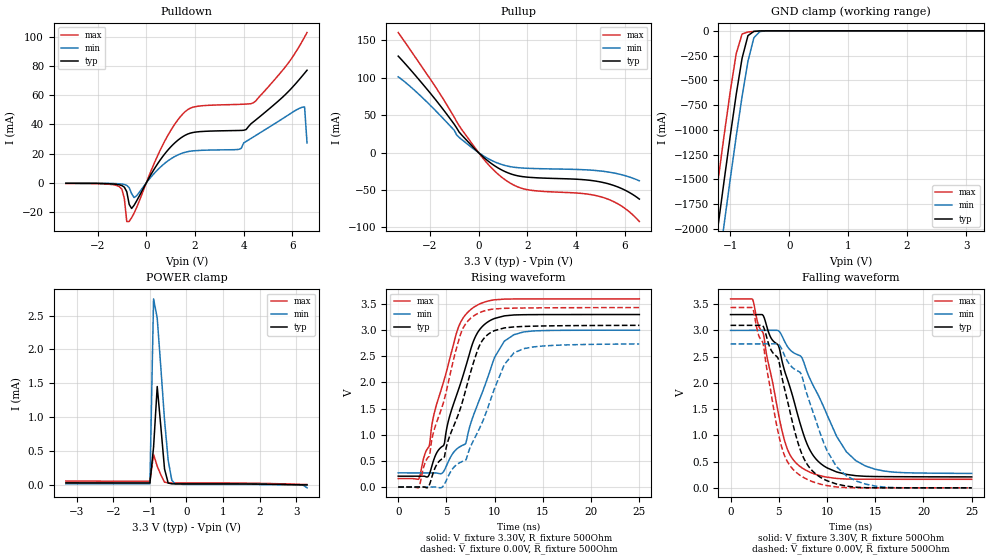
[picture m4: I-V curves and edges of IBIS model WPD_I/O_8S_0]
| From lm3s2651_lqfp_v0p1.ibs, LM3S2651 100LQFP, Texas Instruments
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[Model]   WPD_I/O_8S_0
Model_type   I/O
Vinl = 1.26
Vinh = 2.04
Vmeas = 1.65
| variable   typ   min   max
C_comp   9.739pF   9.739pF   9.739pF
[Model Spec]
Vinh+   1.91   1.78   2.04
Vinh-   1.90   1.76   2.03
Vinl+   1.40   1.27   1.54
Vinl-   1.39   1.26   1.53
| variable   typ   min   max
[Temperature Range]  25   85   -40
[Voltage Range]   3.3V   3.0V   3.6V
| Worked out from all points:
|   slope of the pulldown table from 0 to 0.495 V, typ, clamps not added: 35.8 ohm
|   slope of the pullup table from 0 to 0.495 V, typ, clamps not added: 35.8 ohm
|   GND clamp passes 1 mA (typ) near -0.48 V on its own axis
|   POWER clamp passes 1 mA (typ) near -0.72 V on its own axis
|   falling waveform, V_fixture 3.30V, R_fixture 500Ohm: 20-80 % time 2.93ns typ, 4.09ns min, 2.25ns max; typ from 3.3 V to 0.208 V
|   rising waveform, V_fixture 3.30V, R_fixture 500Ohm: 20-80 % time 2.83ns typ, 3.04ns min, 2.71ns max; typ from 0.208 V to 3.3 V
|   falling waveform, V_fixture 0.00V, R_fixture 500Ohm: 20-80 % time 2.55ns typ, 3.29ns min, 2.08ns max; typ from 3.09 V to 0 V
|   rising waveform, V_fixture 0.00V, R_fixture 500Ohm: 20-80 % time 3.13ns typ, 3.58ns min, 2.86ns max; typ from 0 V to 3.09 V
[Pulldown]
|  Voltage   I(typ)   I(min)   I(max)
-3.3V     -256.5uA   -145.6uA   -364.4uA
-1.1V     -1.273mA   -587.4uA   -2.566mA
-900mV    -2.885mA   -1.061mA   -10.54mA
-800mV    -5.992mA   -1.67mA    -26.39mA
-700mV    -14.71mA   -3.214mA   -26.32mA
-500mV    -15.25mA   -9.999mA   -20.65mA
600mV     16.35mA    11.13mA    23.4mA
1.5V      31.67mA    20.51mA    47.18mA
3.8V      35.87mA    22.99mA    53.71mA
4.4V      41.79mA    31.47mA    54.86mA
6.5V      75.05mA    51.94mA    99.75mA
6.6V      77.06mA    27.41mA    102.8mA
[Pullup]
|  Voltage   I(typ)   I(min)   I(max)
-3.3V     128.9mA    101.3mA    160.4mA
-2V       80.11mA    63.76mA    99.01mA
-1V       37.89mA    29.82mA    47.29mA
-700mV    23.8mA     17.69mA    31.26mA
300mV     -8.861mA   -6.312mA   -12.18mA
1V        -24.01mA   -16.38mA   -34.13mA
1.5V      -30.15mA   -19.7mA    -44.24mA
2V        -32.74mA   -20.87mA   -49.48mA
4.3V      -36.12mA   -22.8mA    -54.74mA
5.1V      -39.81mA   -24.88mA   -59.77mA
5.9V      -48.4mA    -29.75mA   -72.06mA
6.6V      -62.06mA   -37.61mA   -92.08mA
[GND Clamp]
|  Voltage   I(typ)   I(min)   I(max)
-3.3V     -11.72A    -12.12A    -11.3A
-1.4V     -2.845A    -3.285A    -2.387A
-1.3V     -2.39A     -2.831A    -1.93A
-1.2V     -1.938A    -2.38A     -1.478A
-1.1V     -1.494A    -1.934A    -1.036A
-1V       -1.059A    -1.496A    -610.6mA
-900mV    -645mA     -1.069A    -232.9mA
-800mV    -277.1mA   -664.4mA   -31.59mA
-700mV    -48.56mA   -306.6mA   -12.1mA
-600mV    -5.561mA   -70.2mA    -6.281mA
-500mV    -1.172mA   -7.88mA    -2.176mA
3.3V      16.11uA    11.84uA    29.77uA
[POWER Clamp]
|  Voltage   I(typ)   I(min)   I(max)
-3.3V     31.42uA    17.14uA    57.54uA
-1V       30.25uA    16.5uA     55.43uA
-900mV    557.3uA    2.746mA    449.1uA
-800mV    1.452mA    2.463mA    276.5uA
-700mV    854.2uA    1.726mA    147.8uA
-600mV    235.9uA    958.2uA    41.01uA
-500mV    28.31uA    363.4uA    30.71uA
-400mV    16.41uA    67.09uA    29.83uA
-300mV    16.12uA    11.84uA    29.79uA
3.1V      2.408uA    -920.8nA   9.197uA
3.2V      1.227uA    -3.925uA   7.474uA
3.3V      -104.7pA   -42.65uA   5.692uA
[Ramp]
| variable   typ   min   max
dV/dt_f   1.85/2.93n   1.63/4.09n   2.06/2.25n
dV/dt_r   1.85/3.13n   1.64/3.58n   2.06/2.86n
R_load = 500Ohm
[Falling Waveform]
V_fixture = 3.30V
V_fixture_min = 3.00V
V_fixture_max = 3.60V
R_fixture = 500Ohm
|   Time   V(typ)   V(min)   V(max)
0s        3.298V     2.996V     3.597V
2.3ns     3.298V     2.998V     3.585V
3.4ns     3.276V     2.998V     2.936V
5ns       2.692V     2.987V     1.378V
5.6ns     2.229V     2.79V      898.3mV
7.2ns     1.235V     2.517V     407.7mV
9.1ns     502.1mV    1.761V     241.2mV
11ns      302.3mV    979.8mV    178.8mV
13ns      231mV      515.9mV    165.4mV
25ns      208.4mV    274.1mV    162.4mV
[Rising Waveform]
V_fixture = 3.30V
V_fixture_min = 3.00V
V_fixture_max = 3.60V
R_fixture = 500Ohm
|   Time   V(typ)   V(min)   V(max)
0s        207.7mV    271.2mV    162.2mV
2.1ns     207.5mV    270.5mV    146.6mV
3.2ns     232.7mV    270.2mV    771.4mV
4.8ns     840.9mV    326.1mV    2.073V
6.1ns     1.783V     732.4mV    2.98V
7ns       2.303V     833.1mV    3.299V
7.7ns     2.739V     1.319V     3.42V
10ns      3.225V     2.483V     3.58V
12ns      3.291V     2.913V     3.596V
25ns      3.299V     2.999V     3.598V
[Falling Waveform]
V_fixture = 0.00V
V_fixture_min = 0.00V
V_fixture_max = 0.00V
R_fixture = 500Ohm
|   Time   V(typ)   V(min)   V(max)
0s        3.093V     2.739V     3.433V
2.3ns     3.093V     2.74V      3.421V
3.4ns     3.071V     2.74V      2.73V
4.9ns     2.477V     2.739V     1.087V
5.3ns     2.13V      2.643V     778.7mV
7ns       852.9mV    2.223V     266.6mV
8.1ns     406.7mV    1.685V     148.2mV
10ns      135.5mV    708.4mV    42.72mV
12ns      33.41mV    230.5mV    3.849mV
25ns      39.44uV    90.62uV    23.66uV
[Rising Waveform]
V_fixture = 0.00V
V_fixture_min = 0.00V
V_fixture_max = 0.00V
R_fixture = 500Ohm
|   Time   V(typ)   V(min)   V(max)
0s        403.1uV    2.354mV    175.9uV
2.1ns     186.9uV    995.9uV    -14.86mV
3.1ns     -4.815mV   567.3uV    569mV
4.6ns     543.7mV    4.107mV    1.563V
6.4ns     1.478V     468.1mV    2.886V
7.7ns     2.319V     853mV      3.256V
9.1ns     2.885V     1.418V     3.377V
11ns      3.043V     2.342V     3.417V
12ns      3.062V     2.567V     3.421V
25ns      3.092V     2.736V     3.432V
